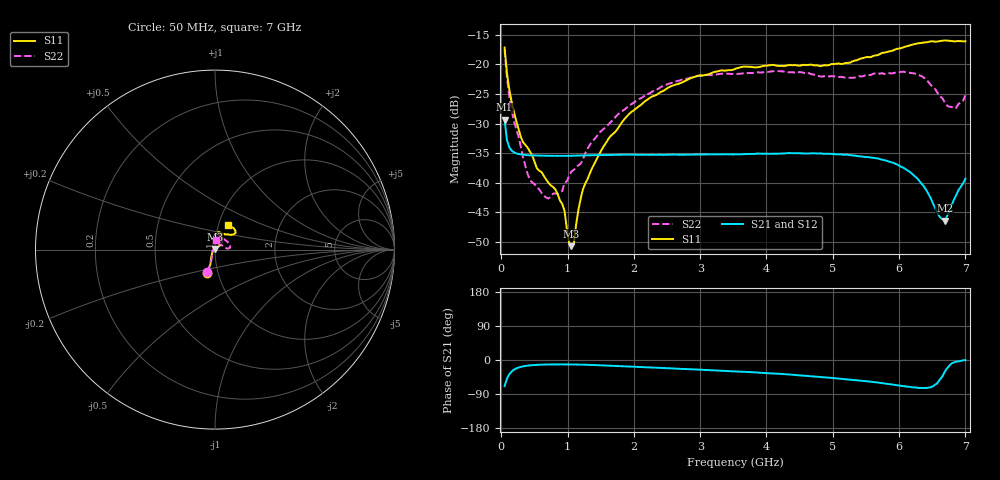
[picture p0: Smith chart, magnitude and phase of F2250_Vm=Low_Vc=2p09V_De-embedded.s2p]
! Integrated Device Technology
! Corporate Headquarters
! 6024 Silver Creek Valley Road
! San Jose, CA 95138  USA
! Phone:  1-408-284-8200
! Toll Free:  1-800-223-1366
! Webpage:  http://www.idt.com/
! Timing and RF Division
! 515 Groton Road, Suite 102
! Westford, MA 01886-6024
! Device:  F2250
! Description: Voltage Variable RF Attenuator
! Frequency:  50.0 -  6000.00 MHz
! Package:  3x3 mm Thin QFN Plastic Package: 16 pin
! Ports:  2 RF, 3 DC
!  Pin  1  = GND
!  Pin  2  = NC
!  Pin  3  = RF1  = Port 1
!  Pin  4  = NC
!  Pin  5  = GND
!  Pin  6  = GND
!  Pin  7  = GND
!  Pin  8  = GND
!  Pin  9  = NC
!  Pin 10  = RF2  = Port 2
!  Pin 11  = NC
!  Pin 12  = GND
!  Pin 13  = GND
!  Pin 14  = VCNTRL
!  Pin 15  = VDD
!  Pin 16  = VMODE
! Vcntrl:  2.090 Volts
! Vmode:  +0.000 Volts
! Vdd:  +3.30  Volts
! Current:  1.180 mA
! Data:  The device was measured on a the F2250 evaluation board which has
!  individual transmission lines to the RF pins.  Data was collected
!  using a calibrated network analyzer.  The evaluation board was
!  de-embedded using a TRL calibration technique.
!  The reference plane is the edge of the package pin.
! Misc:  SN 10
!  Action Tracker AT0258
! Date Measured:  2014-11-26
! Date:  2015-10-15  MJV
! Note:
!  Integrated Device Technology supplies this data as a sample of measured
!  data at the package pin for this product.  Your particular data for this
!  product may vary.
!  Data was taken at 25 degrees C.
!  Integrated Device Technology reserves the right to change this data at anytime.
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# GHz S dB R 50
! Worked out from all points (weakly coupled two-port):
!   201 points, 50 MHz to 7 GHz, reference 50 ohm
!   highest |S21| = -29.34 dB at 50 MHz (marker M1); lowest = -46.4 dB at 6.687 GHz (marker M2)
!   lowest |S11| = -50.7 dB at 1.058 GHz (marker M3), VSWR 1.01, Z = 49.8 + j0.244 ohm
!   |S11| at or under -10 dB: start of sweep to end of sweep
!   |S22| runs from -42.7 to -17.6 dB; largest |S21 - S12| = 5.7e-05
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0.05  -17.18 -108.6  -29.34 -68.9  -29.33 -68.9  -17.57 -109.6
0.08475  -21.44 -107.4  -32.77 -49.6  -32.77 -49.5  -22.18 -106.7
0.189  -28.00 -119.7  -34.85 -25.8  -34.85 -25.8  -29.50 -118.6
0.29325  -32.21 -127.7  -35.21 -18.2  -35.21 -18.2  -33.85 -125.2
0.43225  -34.73 -144.7  -35.37 -14.1  -35.37 -14.1  -39.57 -158.3
0.71025  -39.98 -168.4  -35.45 -11.8  -35.45 -11.8  -42.65 144.4
0.91875  -43.55 158.0  -35.46 -11.6  -35.46 -11.6  -41.39 109.3
0.9535  -44.70 169.8  -35.46 -11.6  -35.46 -11.6  -40.03 109.9
1.023  -50.08 143.7  -35.45 -11.7  -35.45 -11.7  -38.83 91.0
1.05775  -50.69 123.1  -35.45 -11.8  -35.45 -11.8  -38.12 86.5
1.0925  -50.43 89.4  -35.44 -11.9  -35.43 -11.8  -37.81 81.4
1.162  -44.62 56.7  -35.42 -12.0  -35.42 -12.0  -37.05 70.7
1.2315  -41.11 44.2  -35.39 -12.3  -35.39 -12.3  -36.06 62.6
1.6485  -32.11 42.0  -35.31 -14.9  -35.31 -14.9  -29.78 53.2
2.37825  -24.88 47.3  -35.27 -20.7  -35.27 -20.7  -24.08 51.1
3.525  -20.80 72.5  -35.21 -30.1  -35.21 -30.0  -21.66 71.8
4.7065  -20.17 72.4  -35.02 -43.2  -35.03 -43.1  -21.74 70.6
5.85325  -17.82 40.4  -36.44 -63.7  -36.44 -63.8  -21.51 20.0
6.33975  -16.40 41.0  -40.17 -73.8  -40.18 -73.9  -22.02 5.8
6.68725  -15.99 48.8  -46.37 -31.6  -46.35 -31.1  -26.37 25.9
6.82625  -16.13 53.6  -42.87 -6.6  -42.83 -6.5  -27.47 52.8
7  -16.12 63.2  -39.31 -0.5  -39.27 -0.7  -25.22 85.3
